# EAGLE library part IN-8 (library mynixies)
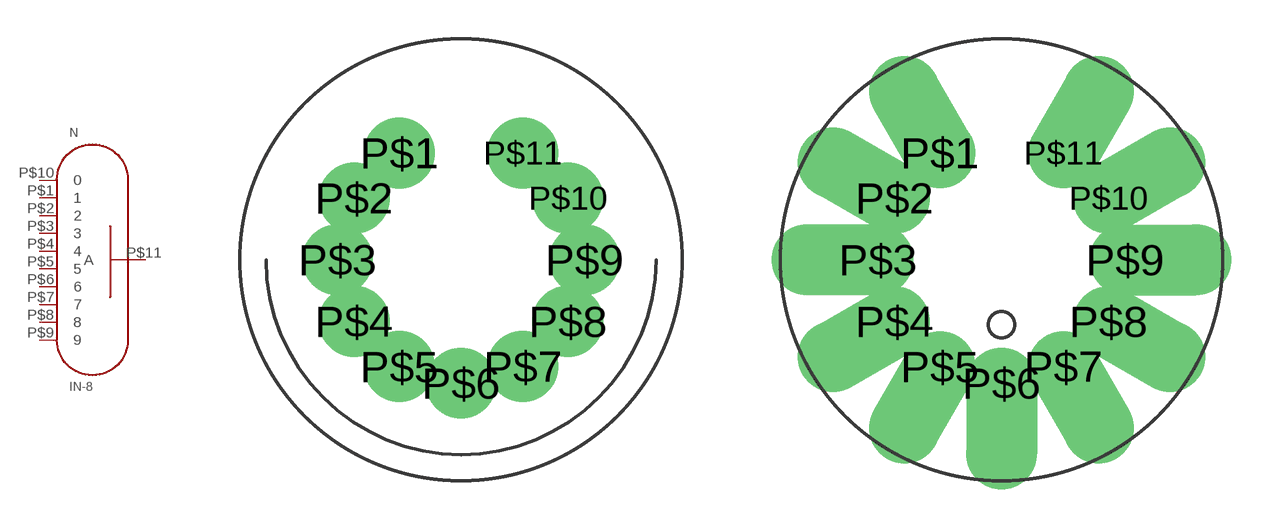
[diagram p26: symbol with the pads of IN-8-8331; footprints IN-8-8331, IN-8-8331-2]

Designator prefix N

## IN-8  [IN-8-8331]
P$1  1  pas
P$2  2  pas
P$3  3  pas
P$4  4  pas
P$5  5  pas
P$6  6  pas
P$7  7  pas
P$8  8  pas
P$9  9  pas
P$10  0  pas
P$11  A  pas

## IN-8L  [IN-8-8331-2]
Pads as for IN-8-8331

## Footprint IN-8-8331 (pad centres in mm)
drill 1.82 pad 2.2: P$1 -2.375,4.114; P$2 -4.114,2.375; P$3 -4.75,0; P$4 -4.114,-2.375; P$5 -2.375,-4.114; P$6 0,-4.75; P$7 2.375,-4.114; P$8 4.114,-2.375; P$9 4.75,0; P$10 4.114,2.375; P$11 2.375,4.114

## Footprint IN-8-8331-2 (pad centres in mm)
drill 1.82 pad 2.2 offset: P$1 -2.375,4.114; P$2 -4.114,2.375; P$3 -4.75,0; P$4 -4.114,-2.375; P$5 -2.375,-4.114; P$6 0,-4.75; P$7 2.375,-4.114; P$8 4.114,-2.375; P$9 4.75,0; P$10 4.114,2.375; P$11 2.375,4.114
